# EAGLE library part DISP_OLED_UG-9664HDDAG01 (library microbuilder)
OLED 96x64 Pixel, 0.95" 65K Color
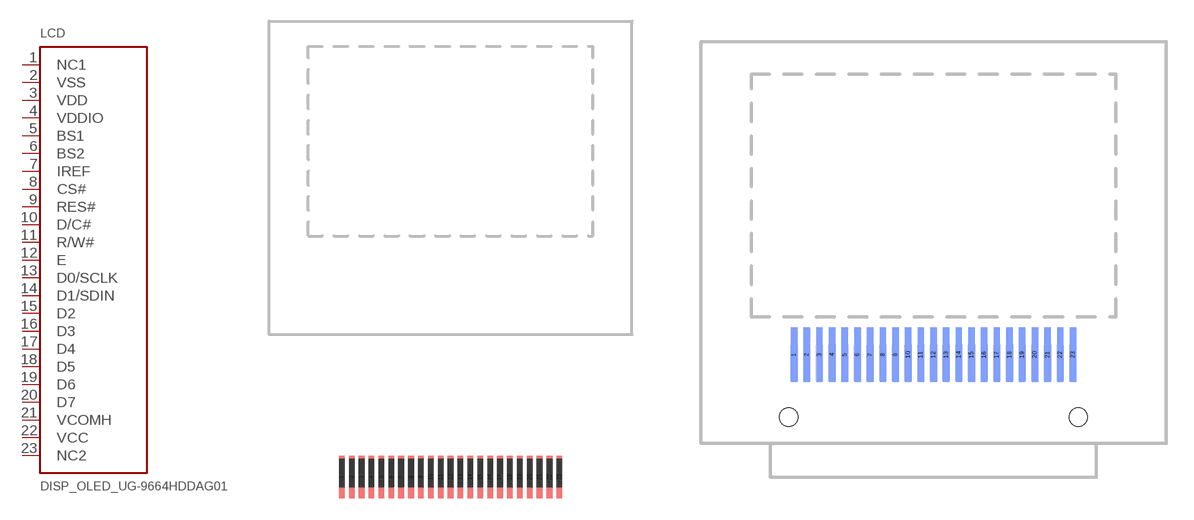
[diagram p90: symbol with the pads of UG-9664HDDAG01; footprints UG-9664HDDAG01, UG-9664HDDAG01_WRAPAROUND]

Designator prefix LCD

## DISP_OLED_UG-9664HDDAG01  [UG-9664HDDAG01]
1  NC1  nc
2  VSS
3  VDD
4  VDDIO
5  BS1
6  BS2
7  IREF
8  CS#
9  RES#
10  D/C#
11  R/W#
12  E
13  D0/SCLK
14  D1/SDIN
15  D2
16  D3
17  D4
18  D5
19  D6
20  D7
21  VCOMH
22  VCC
23  NC2  nc

## DISP_OLED_UG-9664HDDAG01WRAPAROUND  [UG-9664HDDAG01_WRAPAROUND]
Pads as for UG-9664HDDAG01

## DISP_OLED_UG-9664HDDAG01WA_NOHOLES  [UG-9664HDDAG01_WRAPAROUND_NOHOLES]
Pads as for UG-9664HDDAG01

## Footprint UG-9664HDDAG01 (pad centres in mm)
96x64 RGB OLED Display - 0.95" (25.7x22.2mm)
smd 0.4 x 3: 1 -7.7,0.7; 2 -7,0.7; 3 -6.3,0.7; 4 -5.6,0.7; 5 -4.9,0.7; 6 -4.2,0.7; 7 -3.5,0.7; 8 -2.8,0.7; 9 -2.1,0.7; 10 -1.4,0.7; 11 -0.7,0.7; 12 0,0.7; 13 0.7,0.7; 14 1.4,0.7; 15 2.1,0.7; 16 2.8,0.7; 17 3.5,0.7; 18 4.2,0.7; 19 4.9,0.7; 20 5.6,0.7; 21 6.3,0.7; 22 7,0.7; 23 7.7,0.7

## Footprint UG-9664HDDAG01_WRAPAROUND (pad centres in mm)
smd 0.35 x 3 bottom: 1 -7.7,4.9; 2 -7,4.9; 3 -6.3,4.9; 4 -5.6,4.9; 5 -4.9,4.9; 6 -4.2,4.9; 7 -3.5,4.9; 8 -2.8,4.9; 9 -2.1,4.9; 10 -1.4,4.9; 11 -0.7,4.9; 12 0,4.9; 13 0.7,4.9; 14 1.4,4.9; 15 2.1,4.9; 16 2.8,4.9; 17 3.5,4.9; 18 4.2,4.9; 19 4.9,4.9; 20 5.6,4.9; 21 6.3,4.9; 22 7,4.9; 23 7.7,4.9
hole 1 at -8,1.45
hole 1 at 8,1.45

## Footprint UG-9664HDDAG01_WRAPAROUND_NOHOLES (pad centres in mm)
smd 0.35 x 3 bottom: 1 -7.7,4.9; 2 -7,4.9; 3 -6.3,4.9; 4 -5.6,4.9; 5 -4.9,4.9; 6 -4.2,4.9; 7 -3.5,4.9; 8 -2.8,4.9; 9 -2.1,4.9; 10 -1.4,4.9; 11 -0.7,4.9; 12 0,4.9; 13 0.7,4.9; 14 1.4,4.9; 15 2.1,4.9; 16 2.8,4.9; 17 3.5,4.9; 18 4.2,4.9; 19 4.9,4.9; 20 5.6,4.9; 21 6.3,4.9; 22 7,4.9; 23 7.7,4.9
